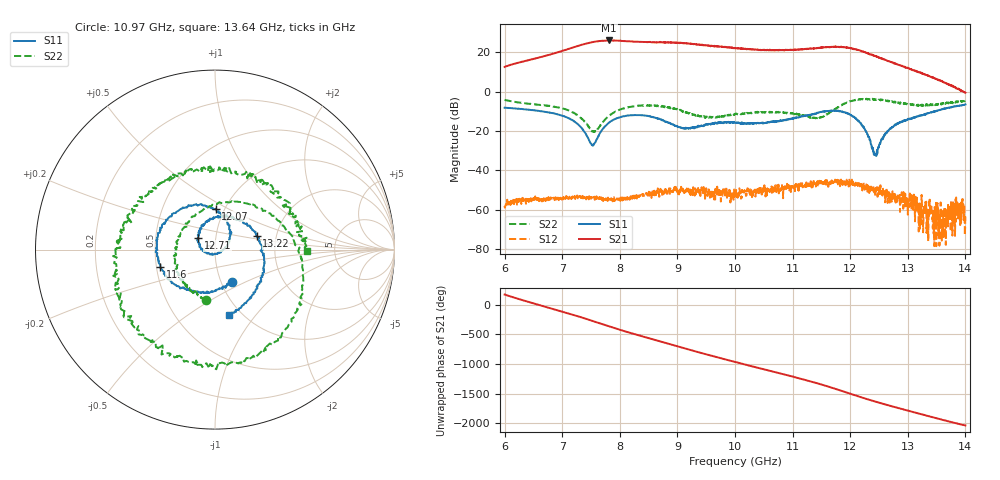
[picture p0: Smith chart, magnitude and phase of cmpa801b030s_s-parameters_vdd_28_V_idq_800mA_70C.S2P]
!Keysight Technologies,E5071C,MY46110325,B.14.03
!Date: Fri Aug 07 15:38:53 2020
!Data & Calibration Information:
!Freq	S11:SOLT2(ON)	S21:SOLT2(ON)	S12:SOLT2(ON)	S22:SOLT2(ON)
!PortZ  Port1:50+j0  Port2:50+j0
!Above PortZ is port z conversion or system Z0 setting when saving the data.
!When reading, reference impedance value at option line is always used.
# Hz S dB R 50
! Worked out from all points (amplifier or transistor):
!   1601 points, 6 GHz to 14 GHz, reference 50 ohm
!   highest |S21| = 26.0 dB at 7.815 GHz (marker M1)
!   |S21| within 3 dB of that: 7.248 GHz to 9.628 GHz (2.38 GHz wide, 28.2 % of centre)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
!   unconditionally stable (mu >= 1): start of sweep to end of sweep
!   at 7.33 GHz: K = 15.82, MAG = 24.0 dB, |S12| = -54.2 dB
!   at 10 GHz: K = 14.27, MAG = 22.6 dB, |S12| = -52.1 dB
!   at 14 GHz: K = 371.45, MAG = 2.4 dB, |S12| = -62.8 dB
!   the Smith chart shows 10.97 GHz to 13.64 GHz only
!   S11 on the Smith chart (normalised r, x): 10.97 GHz: 1.12, -0.43; 11.6 GHz: 0.52, -0.11; 12.07 GHz: 0.91, +0.44; 12.71 GHz: 0.82, +0.11; 13.22 GHz: 1.58, +0.25; 13.64 GHz: 0.88, -0.75
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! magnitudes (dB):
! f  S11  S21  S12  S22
! 6 GHz  -8.2  12.5  -58.2  -4.2
! 6.895 GHz  -11.4  19.7  -54.2  -7.9
! 7.335 GHz  -18.5  23.8  -52.9  -13.7
! 7.535 GHz  -27.0  25.2  -53.8  -20.1
! 7.815 GHz  -15.8  26.0  -54.1  -12.2
! 8.17 GHz  -12.1  25.5  -55.0  -7.8
! 8.67 GHz  -13.8  25.1  -50.9  -7.3
! 9.115 GHz  -19.0  24.7  -52.5  -10.1
! 10 GHz  -15.8  22.1  -52.1  -11.6
! 10.97 GHz  -13.8  21.4  -51.1  -11.0
! 11.34 GHz  -11.7  21.9  -48.8  -13.3
! 11.6 GHz  -9.9  22.5  -45.0  -11.6
! 12.07 GHz  -12.8  21.7  -46.9  -4.5
! 12.27 GHz  -19.8  19.8  -49.5  -3.8
! 12.43 GHz  -31.7  18.0  -48.3  -4.1
! 12.67 GHz  -19.6  15.5  -53.4  -4.6
! 12.71 GHz  -18.9  15.0  -54.4  -5.1
! 13.07 GHz  -13.4  11.1  -58.6  -6.4
! 13.22 GHz  -12.2  9.7  -67.9  -6.8
! 13.64 GHz  -8.5  4.5  -69.4  -5.8
! 13.87 GHz  -7.3  1.3  -60.6  -4.9
! 14 GHz  -6.5  -0.5  -62.8  -4.6
